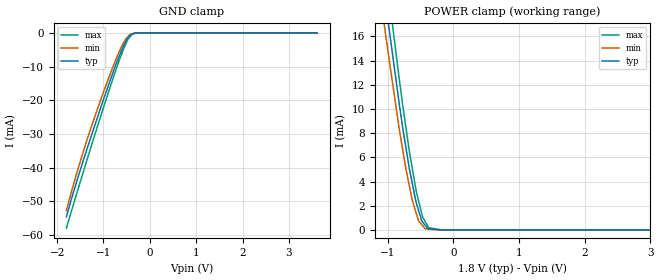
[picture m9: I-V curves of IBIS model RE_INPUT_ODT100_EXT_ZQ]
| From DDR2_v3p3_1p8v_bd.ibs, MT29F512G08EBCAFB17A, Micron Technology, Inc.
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| MODEL RE_INPUT_ODT100_EXT_ZQ (RE Input Model with 100ohm ODT, With ZQ Cal)
[Model]   RE_INPUT_ODT100_EXT_ZQ
Model_type   Input
Vinl = 650.000mV
Vinh = 1.150V
|   typ   min   max
|C_comp   1.146pF   1.033pF   1.260pF
C_comp_power_clamp   0.5730pF   0.5165pF   0.6300pF
C_comp_gnd_clamp   0.5730pF   0.5165pF   0.6300pF
| Note: C_comp changes when the ODT circuit is enabled.
[Model Spec]
| Input threshold voltage corners
Vinl   0.6500V   0.6000V   0.7250V
Vinh   1.1500V   1.1000V   1.2250V
| Dynamic Overshoot Parameters from ONFI4 Specification
D_overshoot_ampl_h   1.00   NA   NA
D_overshoot_ampl_l   1.00   NA   NA
D_overshoot_area_h   0.75n   NA   NA
D_overshoot_area_l   0.75n   NA   NA
[Receiver Thresholds]
|Vth   =  0.900V
|Vth_min  =  0.8820V
|Vth_max  =  0.9180V
|Vinh_ac  =  0.250V
|Vinh_dc  =  0.125V
|Vinl_ac  = -0.250V
|Vinl_dc  = -0.125V
|Tslew_ac =  5.000ns |Not specified, so set to high value
|Threshold_sensitivity = 0.50
|Reference_supply Power_clamp_ref
Vcross_low   = 0.725V
Vcross_high  = 1.075V
Vdiff_ac   = 500mV
Vdiff_dc   = 250mV
Tdiffslew_ac = 10.000ns |Not specified, so set to high value
[Voltage Range]   1.8000V   1.7000V   1.9500V
[POWER Clamp Reference]   1.8000V   1.7000V   1.9500V
| Junction Temperature (Ambient temp is 35C typ, 70C min, 0C max)
[Temperature Range]   50.0   85.0   0.0
[Add Submodel]
| Submodel Name   Mode
100ohm_ODT_EXT_ZQ   Non-Driving
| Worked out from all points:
|   GND clamp passes 1 mA (typ) near -0.44 V on its own axis
|   POWER clamp passes 1 mA (typ) near -0.50 V on its own axis
[GND Clamp]
|   Voltage   I(typ)   I(min)   I(max)
-1.8V     -54.56mA   -52.69mA   -57.93mA
-1.554V   -43.01mA   -40.54mA   -46.59mA
-1.336V   -33.61mA   -30.93mA   -36.81mA
-1.036V   -21.2mA    -18.93mA   -23.66mA
-829.3mV  -13.08mA   -11.23mA   -14.95mA
-630.4mV  -5.889mA   -4.612mA   -7.067mA
-531.8mV  -2.931mA   -2.046mA   -3.69mA
-472.1mV  -1.487mA   -1.111mA   -1.902mA
-431.5mV  -903.3uA   -483.2uA   -1.222mA
-378mV    -285.6uA   -293uA     -327uA
-178.2mV  -2.719uA   -1.561uA   -751.9nA
3.604V    0A         0A         0A
[POWER Clamp]
|   Voltage   I(typ)   I(min)   I(max)
-1.8V     59.37mA    57.52mA    61.9mA
-1.055V   19.69mA    17mA       22.54mA
-1.034V   18.79mA    16.14mA    21.56mA
-829.3mV  10.55mA    8.462mA    12.64mA
-729mV    6.964mA    5.185mA    8.66mA
-630.4mV  3.937mA    2.522mA    5.201mA
-531mV    1.618mA    753.4uA    2.409mA
-472.1mV  669.5uA    367.5uA    1.103mA
-431.5mV  391.1uA    106.3uA    708.2uA
-376.5mV  100.3uA    62.6uA     180.1uA
-178.2mV  0A         501.6nA    561.5nA
3.604V    0A         0A         0A
